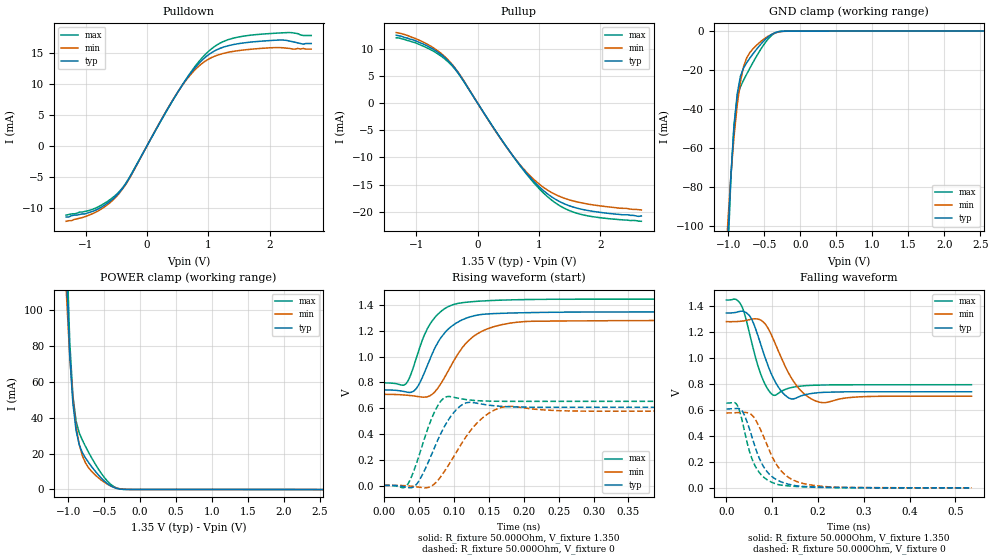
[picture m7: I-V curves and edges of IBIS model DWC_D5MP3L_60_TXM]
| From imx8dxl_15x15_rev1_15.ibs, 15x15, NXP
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[Model] DWC_D5MP3L_60_TXM
Model_type   I/O
Polarity   Non-Inverting
Enable   Active-High
C_comp   1.262pF   1.180pF   1.365pF
C_comp_pullup   279.441fF   258.852fF   306.885fF
C_comp_pulldown 973.651fF   908.565fF   1.053pF
Vinh = 800.000mV
Vinl = 550.000mV
Vmeas = 675.000mV
Vref = 675.000mV
Rref = 50Ohms
Cref = 0pF
[Model Spec]
Vinh   800.000mV   766.500mV   850.000mV
Vinl   550.000mV   516.500mV   600.000mV
Vmeas   675.000mV   641.500mV   725.000mV
Vref   675.000mV   641.500mV   725.000mV
D_overshoot_ampl_h 0.4 NA   NA
D_overshoot_ampl_l 0.4 NA   NA
D_overshoot_area_l 100.000p NA   NA
D_overshoot_area_h 100.000p NA   NA
[Receiver Thresholds]
Vth = 675.000mV
Vth_min = 661.500mV
Vth_max = 688.500mV
Vinh_ac = 125.000mV
Vinh_dc = 90.000mV
Vinl_ac = -125.000mV
Vinl_dc = -90.000mV
Tslew_ac = 5.000ns
Threshold_sensitivity = 0.5
Reference_supply Pullup_ref
[Temperature Range]   25.000   125.000   -40.000
[Voltage Range]   1.350V   1.283V   1.450V
[GND Clamp Reference]   0.00V   0.00V   0.00V
[C Comp Corner]
| variable   typ   min   max
C_comp 1.262pF   1.365pF   1.180pF
C_comp_pullup 279.441fF   306.885fF   258.852fF
C_comp_pulldown 973.651fF   1.053pF   908.565fF
[Pulldown Reference]   0.00V   0.00V   0.00V
[POWER Clamp Reference]   1.350V   1.283V   1.450V
[Pullup Reference]   1.350V   1.283V   1.450V
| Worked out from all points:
|   slope of the pulldown table from 0 to 0.203 V, typ, clamps not added: 55.7 ohm
|   slope of the pullup table from 0 to 0.203 V, typ, clamps not added: 56.7 ohm
|   GND clamp passes 1 mA (typ) near -0.36 V on its own axis
|   POWER clamp passes 1 mA (typ) near -0.36 V on its own axis
|   rising waveform, R_fixture 50.000Ohm, V_fixture 1.350: 20-80 % time 37.8ps typ, 45.4ps min, 32.2ps max; typ from 0.742 V to 1.35 V
|   rising waveform, R_fixture 50.000Ohm, V_fixture 0: 20-80 % time 31.1ps typ, 41.9ps min, 24.5ps max; typ from 0.001 V to 0.608 V
|   falling waveform, R_fixture 50.000Ohm, V_fixture 1.350: 20-80 % time 36.5ps typ, 46.5ps min, 28.6ps max; typ from 1.35 V to 0.74 V
|   falling waveform, R_fixture 50.000Ohm, V_fixture 0: 20-80 % time 42.3ps typ, 50.9ps min, 35.1ps max; typ from 0.608 V to 0 V
[GND Clamp]
-1.318V   -593.4mA   -427mA     -758.7mA
-1.011V   -108.7mA   -99.8mA    -118.2mA
-966.7mV  -74.7mA    -74.6mA    -75.87mA
-922.7mV  -49.41mA   -54.3mA    -47.9mA
-878.8mV  -32.42mA   -38.21mA   -34.12mA
-834.8mV  -23.33mA   -26.23mA   -28.72mA
-790.9mV  -19.01mA   -18.35mA   -25.26mA
-747mV    -16.25mA   -13.76mA   -22.11mA
-483.3mV  -4.093mA   -3.434mA   -5.633mA
-351.5mV  -766.8uA   -911.3uA   -894.7uA
-263.6mV  -79.41uA   -192.1uA   -51.43uA
2.68V     154.9uA    127.3uA    193.1uA
[Power Clamp]
-1.33V    727.8mA    510.6mA    954.1mA
-1.023V   119.4mA    107.4mA    137.5mA
-978.8mV  74.87mA    74.2mA     82.23mA
-934.8mV  47.95mA    50.66mA    52.21mA
-890.9mV  32.9mA     35.12mA    38.1mA
-847mV    24.9mA     25.11mA    31.53mA
-759.1mV  17.5mA     14.71mA    23.9mA
-671.2mV  12.54mA    9.915mA    17.38mA
-495.5mV  4.603mA    3.922mA    6.563mA
-363.6mV  1.088mA    1.21mA     1.541mA
-231.8mV  46.56uA    141.4uA    53.69uA
2.668V    -76.24uA   -66.58uA   -87.76uA
[Pulldown]
-1.318V   -11.5mA    -12.2mA    -11.2mA
-834.8mV  -10.39mA   -10.73mA   -10.05mA
-615.2mV  -9.06mA    -9.294mA   -8.789mA
-439.4mV  -7.411mA   -7.525mA   -7.263mA
-307.6mV  -5.543mA   -5.636mA   -5.466mA
483.3mV   8.402mA    8.419mA    8.395mA
703mV     11.64mA    11.45mA    11.77mA
922.7mV   14.12mA    13.55mA    14.53mA
1.186V    15.79mA    14.83mA    16.63mA
1.494V    16.58mA    15.45mA    17.66mA
2.197V    17.17mA    15.93mA    18.33mA
2.68V     16.6mA     15.7mA     17.9mA
[Pullup]
-1.33V    12.6mA     13.1mA     12.13mA
-803mV    10.5mA     10.82mA    10.13mA
-627.3mV  9.274mA    9.502mA    8.976mA
-451.5mV  7.529mA    7.658mA    7.332mA
-275.8mV  4.943mA    5.041mA    4.864mA
207.6mV   -3.657mA   -3.719mA   -3.635mA
559.1mV   -9.476mA   -9.478mA   -9.507mA
822.7mV   -13.27mA   -13.03mA   -13.46mA
1.086V    -16.26mA   -15.64mA   -16.72mA
1.35V     -18.24mA   -17.27mA   -19.01mA
1.658V    -19.48mA   -18.31mA   -20.44mA
2.668V    -20.8mA    -19.7mA    -21.8mA
[Ramp]
R_load=50.000Ohm
dV/dt_r   364.350mV/35.500ps  345.537mV/45.000ps  391.320mV/29.500ps
dV/dt_f   364.350mV/40.500ps  345.537mV/50.000ps  391.290mV/33.000ps
[Rising waveform]
R_fixture=50.000Ohm
V_fixture=1.350
V_fixture_min=1.283
V_fixture_max=1.450
0s        742.1mV    707.8mV    796.7mV
30ps      728.5mV    702.6mV    783.9mV
44ps      739.4mV    694.3mV    949.3mV
56ps      851.5mV    686mV      1.144V
69ps      1.022V     708.2mV    1.278V
85ps      1.173V     822.4mV    1.366V
105ps     1.266V     1.014V     1.413V
133ps     1.322V     1.176V     1.43V
189ps     1.34V      1.267V     1.442V
535ps     1.348V     1.281V     1.447V
[Rising waveform]
R_fixture=50.000Ohm
V_fixture=0
0s        1.203mV    1.231mV    1.012mV
33ps      -14.86mV   -2.014mV   1.732mV
50ps      35.33mV    -13.32mV   228.3mV
72ps      290.1mV    10.98mV    567.2mV
90ps      490.1mV    137.9mV    689.6mV
104ps     591.3mV    261.5mV    680.2mV
118ps     642mV      383mV      666.7mV
144ps     628.3mV    537.6mV    656.1mV
172ps     613.2mV    611mV      653.5mV
535ps     608.2mV    577.3mV    654mV
[Falling waveform]
R_fixture=50.000Ohm
V_fixture=1.350
V_fixture_min=1.283
V_fixture_max=1.450
0s        1.347V     1.281V     1.447V
29ps      1.359V     1.283V     1.427V
38ps      1.359V     1.286V     1.361V
50ps      1.329V     1.295V     1.199V
77ps      1.084V     1.289V     858.1mV
103ps     842mV      1.142V     714mV
140ps     687.2mV    858.1mV    771.2mV
167ps     712.9mV    733.6mV    785.7mV
200ps     733mV      663.2mV    791.5mV
535ps     740.4mV    706.3mV    794.6mV
[Falling waveform]
R_fixture=50.000Ohm
V_fixture=0
0s        607.5mV    577mV      652.6mV
18ps      610.7mV    578.7mV    657.1mV
25ps      611.9mV    579.8mV    628.1mV
38ps      571.7mV    581.5mV    464.2mV
57ps      381.2mV    556.9mV    214.6mV
79ps      176.8mV    413.8mV    90.32mV
107ps     68.33mV    193.9mV    31.56mV
140ps     24.48mV    71.3mV     13.67mV
192ps     7.39mV     18.52mV    4.4mV
535ps     16.32uV    101.6uV    7.984uV
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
